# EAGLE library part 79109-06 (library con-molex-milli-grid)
RECEPTACAL
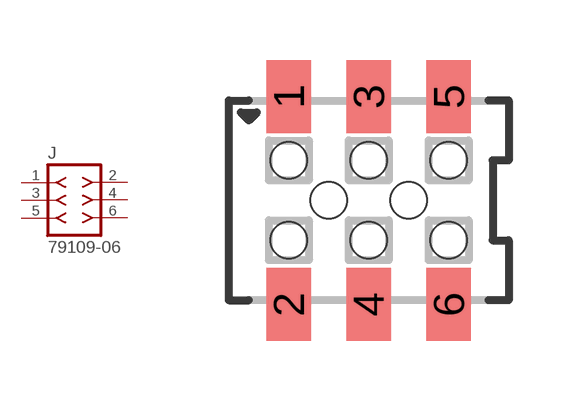
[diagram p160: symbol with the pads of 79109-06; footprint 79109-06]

Designator prefix J

## 79109-06  [79109-06]
1  1  pas
2  2  pas
3  3  pas
4  4  pas
5  5  pas
6  6  pas

## Footprint 79109-06 (pad centres in mm)
RECEPTACAL SMD Dual Row, Vertical, Pass-Thru
smd 1.12 x 1.83: 1 -2,2.6; 2 -2,-2.6; 3 0,2.6; 4 0,-2.6; 5 2,2.6; 6 2,-2.6
hole 0.914 at -1,0
hole 0.914 at -2,1
hole 0.914 at -2,-1
hole 0.914 at 0,-1
hole 0.914 at 0,1
hole 0.914 at 2,-1
hole 0.914 at 2,1
hole 0.914 at 1,0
